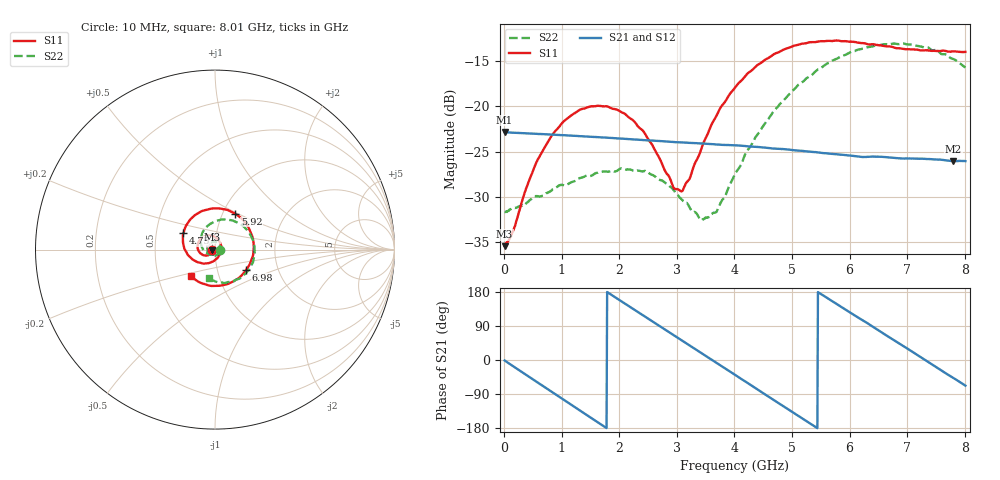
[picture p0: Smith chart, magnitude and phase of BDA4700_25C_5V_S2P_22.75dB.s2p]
!Agilent Technologies,E5071B,MY42404982,A.09.10
!Date: Mon Oct 20 13:37:51 2025
!Data & Calibration Information:
!Freq	S11:SOLT2(ON)	S21:SOLT2(ON)	S12:SOLT2(ON)	S22:SOLT2(ON)
# Hz S RI R 50
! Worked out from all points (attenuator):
!   801 points, 10 MHz to 8.01 GHz, reference 50 ohm
!   highest |S21| = -22.83 dB at 10 MHz (marker M1); lowest = -26.1 dB at 7.8 GHz (marker M2)
!   lowest |S11| = -35.4 dB at 10 MHz (marker M3), VSWR 1.03, Z = 48.3 - j0.108 ohm
!   |S11| at or under -10 dB: start of sweep to end of sweep
!   |S22| runs from -32.6 to -13.0 dB; largest |S21 - S12| = 0.00058
!   S11 on the Smith chart (normalised r, x): 10 MHz: 0.97, -0.00; 4.75 GHz: 0.69, +0.13; 5.92 GHz: 1.14, +0.48; 6.98 GHz: 1.37, -0.33; 8.01 GHz: 0.73, -0.22
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1e7  -0.0169 -0.00111  0.0722 -0.00153  0.0722 -0.00162  0.0261 -0.00083
1.5e8  -0.018 -0.00945  0.069 -0.0193  0.069 -0.0193  0.0263 -0.00712
4.3e8  -0.0285 -0.026  0.051 -0.0494  0.0509 -0.0494  0.0196 -0.0226
7e8  -0.0489 -0.0331  0.0225 -0.0666  0.0225 -0.0665  0.00592 -0.0322
1.02e9  -0.0784 -0.0231  -0.0162 -0.0675  -0.0163 -0.0675  -0.0161 -0.0331
1.35e9  -0.0966 0.00725  -0.0498 -0.047  -0.0498 -0.0471  -0.0364 -0.0177
2.09e9  -0.0481 0.0777  -0.0572 0.0336  -0.0572 0.0336  -0.029 0.0345
2.68e9  0.0238 0.0475  -0.00152 0.0645  -0.0015 0.0645  0.0135 0.0372
2.95e9  0.0343 0.00849  0.027 0.0576  0.0271 0.0575  0.0257 0.0227
3.1e9  0.0309 -0.0149  0.0406 0.0485  0.0405 0.0487  0.0284 0.0107
3.41e9  0.00145 -0.0564  0.0588 0.0212  0.0589 0.0211  0.0203 -0.0123
3.54e9  -0.0179 -0.0687  0.0618 0.0076  0.0618 0.00744  0.0126 -0.0209
3.7e9  -0.0481 -0.0764  0.0609 -0.00927  0.061 -0.00944  -0.00112 -0.0266
4.01e9  -0.1098 -0.0637  0.0474 -0.0385  0.0474 -0.0385  -0.033 -0.0261
4.75e9  -0.1755 0.0925  -0.022 -0.0541  -0.0218 -0.0542  -0.0795 0.0594
5.35e9  -0.0642 0.2175  -0.0554 -0.0088  -0.0555 -0.00894  -0.015 0.1491
5.92e9  0.1123 0.2004  -0.0372 0.039  -0.0373 0.0389  0.1133 0.1558
6.68e9  0.2137 -0.0197  0.0255 0.0456  0.0257 0.0457  0.2204 -0.00154
6.98e9  0.1734 -0.1135  0.0437 0.0276  0.0438 0.0273  0.2052 -0.0818
7.39e9  0.0603 -0.1942  0.0508 -0.00678  0.0508 -0.0069  0.1302 -0.1638
7.8e9  -0.0787 -0.1858  0.0338 -0.0366  0.0337 -0.0367  0.0183 -0.1818
8.01e9  -0.1364 -0.1468  0.019 -0.0461  0.019 -0.0463  -0.0322 -0.1607
